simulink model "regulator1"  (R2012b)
settings: Solver=ode45  StartTime=0.0  StopTime=100.0  MaxStep=0.01  RelTol=1e-3
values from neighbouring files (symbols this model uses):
  hy = 0.01    [fuellstnd_3.m]    (also in fuellstnd_31.m; regulator_1.m = 2; zweipunkt_1.m = 20; zweipunkt_2.m = 0)
  Kr = 2000    [aktiv_tilger_2.m]    (also in beobachter_22.m = 5; fuellstnd_3.m = 10,; fuellstnd_31.m = 10,; kalman_12.m = Kn(1:2))
  Th = 1    [fuellstnd_3.m]    (also in fuellstnd_31.m; regulator_1.m = 10; zweipunkt_31.m = 100; zweipunkt_32.m = 100)
  Tp = 1    [fuellstnd_2.m]    (also in fuellstnd_21.m = 0.1; fuellstnd_3.m = 0.1; fuellstnd_31.m = 0.01; regulator_1.m = 5)
  Ui = 5    [regulator_1.m]
libraries: dspstat3 x2

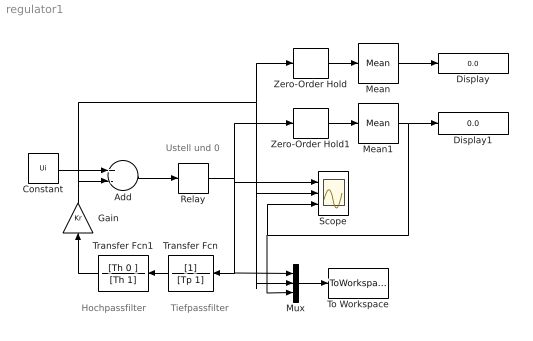
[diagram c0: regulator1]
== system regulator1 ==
  note: Hochpassfilter
  note: Tiefpassfilter
  note: Ustell und 0
  Add : Sum  Inputs=+-
  Constant : Constant  Value=Ui
  Display : Display
  Display1 : Display
  Gain : Gain  Gain=Kr
  Mean : dspstat3/Mean  run=on  reset_popup=None  InputProcessing=Columns as channels (frame based)  directionMode=Each column  dimension=1  treatSBRowAsCol=on  roiEnable=off  roiType=Rectangles  roiPortion=Entire ROI  roiOutput=Individual statistics for each ROI  roiFlag=off  outputDataTypeStr=Inherit: Same as accumulator  outputLastDataTypeStr=Inherit: Same as accumulator  outputMin=[]  outputMax=[]  roundingMode=Floor  overflowMode=off
  Mean1 : dspstat3/Mean  run=on  reset_popup=None  InputProcessing=Columns as channels (frame based)  directionMode=Each column  dimension=1  treatSBRowAsCol=on  roiEnable=off  roiType=Rectangles  roiPortion=Entire ROI  roiOutput=Individual statistics for each ROI  roiFlag=off  outputDataTypeStr=Inherit: Same as accumulator  outputLastDataTypeStr=Inherit: Same as accumulator  outputMin=[]  outputMax=[]  roundingMode=Floor  overflowMode=off
  Mux : Mux  Inputs=3
  Relay : Relay  OnSwitchValue=hy  OffSwitchValue=-hy  OnOutputValue=Ustell
  Scope : Scope  NumInputPorts=3
  To Workspace : ToWorkspace  VariableName=y  SampleTime=-1  SaveFormat=Structure With Time
  Transfer Fcn : TransferFcn  Denominator=[Tp 1]
  Transfer Fcn1 : TransferFcn  Numerator=[Th 0 ]  Denominator=[Th 1]
  Zero-Order Hold : ZeroOrderHold  SampleTime=0.01
  Zero-Order Hold1 : ZeroOrderHold  SampleTime=0.01
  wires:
  Add/1 -> Relay/1
  Relay/1 -> Zero-Order Hold1/1, Mux/1, Transfer Fcn/1, Scope/1
  Constant/1 -> Add/1
  Mean/1 -> Display/1
  Zero-Order Hold/1 -> Mean/1
  Mux/1 -> To Workspace/1
  Gain/1 -> Add/2, Zero-Order Hold/1, Mux/2, Scope/2
  Transfer Fcn/1 -> Transfer Fcn1/1
  Transfer Fcn1/1 -> Gain/1
  Mean1/1 -> Mux/3, Scope/3, Display1/1
  Zero-Order Hold1/1 -> Mean1/1
